PROGRAM MAIN
VAR
	bExecute				: BOOL:=TRUE;
	sRemoteHost				: STRING(15);
	nRemotePort				: UDINT;
	asduAddr				: DWORD;
	nOrgAdd					: BYTE;

	eComState				: E_ComState	:= INIT;
	fbConnection			: FB_ClientServerConnection;
	fbProtocol				: FB_IEC870_5_104TProtocol;
	stBuffer				: ST_IEC870_5_101TBuffer;
	fbBuffer				: FB_IEC870_5_101TBufferCtrl;
	
	stTxAsdu 				: ST_IEC870_5_101AOGen; // Asdu to send 
	stRxAsdu 				: ST_IEC870_5_101AOGen; // Received asdu 
	
	// general interrogation
	bGenInro				: BOOL := TRUE; 	// enable general interrogation
	tGenInro				: TIME := T#20S;	// general interrogation cycle time
	nQOI_GenInro			: BYTE := INT_TO_BYTE(eIEC870_QOI_INROGEN); // qualifier of general interrogation command
	fbGenInroTimer			: TON;
	
	// interrogation group 1
	bInroGrp1				: BOOL := TRUE;		// enable interrogation group 1
	tInroGrp1				: TIME := T#10S;	// interrogation group 1 cycle time
	nQOI_InroGrp1			: BYTE := INT_TO_BYTE(eIEC870_QOI_INRO1);
	fbInroGrp1Timer			: TON;
	// spontaneous data transmission
	fbSpontTime				: TON;
	
END_VAR

// timer
fbSpontTime(IN:= TRUE XOR fbSpontTime.Q, PT:= T#5S);
fbGenInroTimer(IN:= bGeninro XOR fbGenInroTimer.Q, PT:= tGenInro);
fbInroGrp1Timer	(IN:=bInroGrp1 XOR fbInroGrp1Timer.Q, PT:= tInroGrp1);

// connection management
CASE eComState OF
INIT: 
	// TCP/IP connection
	sRemoteHost	:= '127.0.0.1';	// ip-address (slave)
	nRemotePort	:= 2404;			// communication port - check firewall settings
	asduAddr	:= 3;
	nOrgAdd		:= 1;
	
	
	// INIT protocol parameter
	fbConnection.nMode 		:= CONNECT_MODE_ENABLEDBG; // enable debug messages

	fbProtocol.sSrvNetID				:= '';		
	fbProtocol.protPara.sRemoteHost		:= sRemoteHost;	// slave IP-address
	fbProtocol.protPara.nRemotePort		:= nRemotePort;
	fbProtocol.protPara.bControlDT		:= TRUE;	// data transmission controlled by master - ON
	fbProtocol.protPara.bDTControlled 	:= FALSE;	// data transmission controlled by slave - OFF

	fbProtocol.protPara.bPackFrames		:= TRUE;
	fbProtocol.protPara.bThrottleMode	:= TRUE;
	fbProtocol.bOutDbg					:= FALSE;	// disable debug output


	// INIT RX/TX buffer parameter
	stBuffer.eDbg					:= eIEC870_FIFO_DBG_OFF;		// fifo debug off
	stBuffer.asduFmt.eCOTSize		:= eIEC870_COT_TwoOctets;		// cause of transfer size
	stBuffer.asduFmt.eAsduAddrSize	:= eIEC870_AsduAddr_TwoOctets;	// common asdu addr size
	stBuffer.asduFmt.eObjAddrSize	:= eIEc870_ObjAddr_ThreeOctets;	// object address size

	eComState := IDLE;
	
	
IDLE:	
	IF bExecute THEN
		stBuffer.asduSize := F_iecApdu104ToAsduLen(fbProtocol.protPara.APDULength);
		eComState := CONNECT;
	END_IF

	
CONNECT: ;
	fbConnection( 	bEnable := bExecute,
					sRemoteHost	:= fbProtocol.protPara.sRemoteHost,
					nRemotePort	:= fbProtocol.protPara.nRemotePort,
					tReconnect 	:= fbProtocol.protPara.t0 );

	CASE fbConnection.eState OF 
	eSOCKET_CONNECTED:
		fbProtocol.INIT( 	hSocket := fbConnection.hSocket,
							buffer := stBuffer );
		eComState := DATATRANSFER;			
	eSOCKET_DISCONNECTED:
		eComState := IDLE;	
	eSOCKET_SUSPENDED:
		; // wait for connection	
	END_CASE		
		

DATATRANSFER: ;
	IF bExecute THEN
		fbProtocol(buffer := stBuffer);
		IF NOT fbProtocol.bError THEN
			IF fbProtocol.eDTState = eIEC870_STARTDT THEN
				;// exchange data
			END_IF
		ELSE // error occured - log error msg. and close socket
			ADSLOGSTR(	ADSLOG_MSGTYPE_ERROR OR ADSLOG_MSGTYPE_LOG,		// log errors
						'IEC60870-5-104 Transport Interface error: %s',
						DWORD_TO_HEXSTR(fbProtocol.nErrID,0,TRUE));
			eComState := CLOSESOCKEt;
		END_IF
	ELSE // stop data transfer
		fbProtocol.STOPDT(buffer := stBuffer);
		eComState := STOPDATATRANSFER;
	END_IF

	
STOPDATATRANSFER: 
	fbProtocol(buffer := stBuffer);
	IF fbProtocol.eDTState = eIEC870_STOPDT THEN
		eComState := CLOSESOCKET;	// close connection
	END_IF


CLOSESOCKET: ;
	fbConnection(bEnable := FALSE);
	IF fbConnection.eState = eSOCKET_DISCONNECTED THEN
		eComState := IDLE;
	END_IF
END_CASE


// -----------------------------------------------------------------------------------
// process received data

REPEAT
	fbBuffer.RxRemoveObj(	getObj => stRxAsdu,
 							buffer := stBuffer);
								
	IF fbBuffer.bOk THEN
		CASE stRxAsdu.ident.eType OF
		M_SP_NA_1:	// single point without time tag
			CASE stRxAsdu.info.objAddr OF 	
			10: // bSlaveToMaster
				F_iecMoveStreamToBuffer (ADR(nSIQ_bSlaveToMaster),SIZEOF(nSIQ_bSlaveToMaster), stRxAsdu.info.stream); //Copy value to local varialbe
							
				bSlaveToMaster		:= nSIQ_bSlaveToMaster.0;
				eSPI_bSlaveToMaster	:= BOOL_TO_INT(nSIQ_bSlaveToMaster.0);
				nQDS_bSlaveToMaster := SHR((nSIQ_bSlaveToMaster AND 2#1111_0000),4);
			
			ELSE 
				// code for invalid object address
				EXIT; 
			END_CASE
			
		M_BO_NA_1:	// bitstring (32Bit)
			CASE stRxAsdu.info.objAddr OF 	
			11: // nBitstring
				F_iecMoveStreamToBuffer (ADR(nBitstring),SIZEOF(nBitstring), stRxAsdu.info.stream); //Copy value to local varialbe
				F_iecMoveStreamToBuffer (ADR(nQDS_nBitstring),SIZEOF(nQDS_nBitstring), stRxAsdu.info.stream);			
			ELSE 
				// code for invalid object address
				EXIT; 
			END_CASE
		
		M_ME_NB_1:	// measured value (scaled)
			CASE stRxAsdu.info.objAddr OF 	
			12: // nMeasurementValue
				F_iecMoveStreamToBuffer (ADR(nMeasurementValue),SIZEOF(nMeasurementValue), stRxAsdu.info.stream); //Copy value to local varialbe
				F_iecMoveStreamToBuffer (ADR(nQDS_nMeasurementValue),SIZEOF(nQDS_nMeasurementValue), stRxAsdu.info.stream);			
			ELSE 
				// code for invalid object address
				EXIT; 
			END_CASE
		
		M_ME_NC_1:	// measured value (floating point)
			CASE stRxAsdu.info.objAddr OF 	
			13: // fMeasurementValue
				F_iecMoveStreamToBuffer (ADR(fMeasurementValue),SIZEOF(fMeasurementValue), stRxAsdu.info.stream); //Copy value to local varialbe
				F_iecMoveStreamToBuffer (ADR(nQDS_fMeasurementValue),SIZEOF(nQDS_fMeasurementValue), stRxAsdu.info.stream);	
			ELSE 
				// code for invalid object address
				EXIT; 
			END_CASE
		
		ELSE
			// code for invalid asdu types
			EXIT;
		END_CASE
	END_IF

UNTIL NOT fbBuffer.bOk // RX fifo is empty
END_REPEAT


// -----------------------------------------------------------------------------------
// send data

IF fbProtocol.eDTState = eIEC870_STARTDT THEN

	// general interrogation
	IF fbGenInroTimer.Q THEN

		// create asdu
		stTxAsdu.ident.eType	:= C_IC_NA_1;		// interrogation command
		stTxAsdu.info.objAddr	:= 0;				// object address
		stTxAsdu.ident.asduAddr	:= asduAddr;		// common ASDU address
		stTxAsdu.ident.bSQ		:= FALSE;			// sequence - always false
		stTxAsdu.ident.nObj		:= 1;				// number of objects
		stTxAsdu.ident.eCOT		:= eIEC870_COT_ACT;	// cause of transmission - command activation
		stTxAsdu.ident.nORG		:= nOrgAdd;			// originator address
		stTxAsdu.ident.bPN		:= FALSE;			// positive/negative confirmation flag
		stTxAsdu.ident.bT		:= FALSE;			// test flag - not used
		stTxAsdu.ident.eClass	:= eIEC870_Class_1; // priority class

		F_iecResetStream(0,stTxAsdu.info.stream);
		F_iecCopyBufferToStream(ADR(nQOI_GenInro),SIZEOF(nQOI_GenInro), stTxAsdu.info.stream);	// copy values TO transmit stream	
		fbBuffer.TxAddObj(	putObj := stTxAsdu,
							buffer := stBuffer);
				
		IF NOT fbBuffer.bOk THEN
			// code for buffer overflow
			RETURN; 
		END_IF
	END_IF

	// interrogation group 1
	IF fbInroGrp1Timer.Q THEN
	// create asdu
		stTxAsdu.ident.eType	:= C_IC_NA_1;		// interrogation command
		stTxAsdu.info.objAddr	:= 0;				// object address
		stTxAsdu.ident.asduAddr	:= asduAddr;		// common ASDU address
		stTxAsdu.ident.bSQ		:= FALSE;			// sequence - always false
		stTxAsdu.ident.nObj		:= 1;				// number of objects
		stTxAsdu.ident.eCOT		:= eIEC870_COT_ACT;	// cause of transmission - command activation
		stTxAsdu.ident.nORG		:= nOrgAdd;			// originator address
		stTxAsdu.ident.bPN		:= FALSE;			// positive/negative confirmation flag
		stTxAsdu.ident.bT		:= FALSE;			// test flag - not used
		stTxAsdu.ident.eClass	:= eIEC870_Class_1; // priority class

		F_iecResetStream(0,stTxAsdu.info.stream);
		F_iecCopyBufferToStream(ADR(nQOI_InroGrp1),SIZEOF(nQOI_InroGrp1), stTxAsdu.info.stream);	// copy values TO transmit stream	
		fbBuffer.TxAddObj(	putObj := stTxAsdu,
							buffer := stBuffer);
				
		IF NOT fbBuffer.bOk THEN
			// code for buffer overflow
			RETURN; 
		END_IF
	END_IF
	
	// send command on timer expiration or when command data value changes
	IF fbSpontTime.Q OR_ELSE (nSCO_bMasterToSlave.0 <> bMasterToSlave) THEN
		// send single commmands - C_SC_NA_1
	
		//bMasterToSlave	
		nSCO_bMasterToSlave.0	:= bMasterToSlave;
		eSCS_bMasterToSlave		:= BOOL_TO_INT(bMasterToSlave);
		nSCO_bMasterToSlave		:= nSCO_bMasterToSlave OR SHL(INT_TO_BYTE(eQU_bMasterToSlave),2);
		nSCO_bMasterToSlave.7	:= 0;// set S/E bit, 0 -> Execute, 1 -> Select.
		
		// create asdu - bMasterToSlave
		stTxAsdu.ident.eType	:= C_SC_NA_1;		// single command without time tag
		stTxAsdu.info.objAddr	:= 101;				// objecct address
		stTxAsdu.ident.asduAddr	:= asduAddr;		// common ASDU address
		stTxAsdu.ident.bSQ		:= FALSE;			// sequence - always false
		stTxAsdu.ident.nObj		:= 1;				// number of objects
		stTxAsdu.ident.eCOT		:= eIEC870_COT_ACT;	// cause of transmission - spontaneous
		stTxAsdu.ident.nORG		:= nOrgAdd;			// originator address
		stTxAsdu.ident.bPN		:= FALSE;			// positive/negative confirmation flag
		stTxAsdu.ident.bT		:= FALSE;			// test flag - not used
		stTxAsdu.ident.eClass	:= eIEC870_Class_1; // priority class
		
		F_iecResetStream(0,stTxAsdu.info.stream);
		F_iecCopyBufferToStream(ADR(nSCO_bMasterToSlave),SIZEOF(nSCO_bMasterToSlave), stTxAsdu.info.stream);		
		fbBuffer.TxAddObj(	putObj := stTxAsdu,
							buffer := stBuffer);
							
		IF NOT fbBuffer.bOk THEN
			// code for buffer overflow
			RETURN; 
		END_IF						
	
	END_IF	
END_IF

END_PROGRAM
